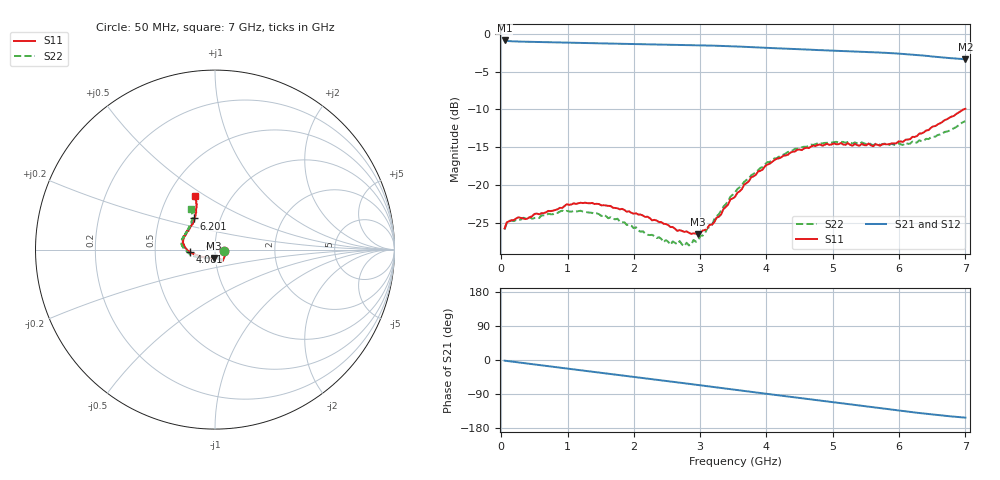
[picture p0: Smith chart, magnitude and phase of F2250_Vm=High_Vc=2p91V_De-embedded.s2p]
! Integrated Device Technology
! Corporate Headquarters
! 6024 Silver Creek Valley Road
! San Jose, CA 95138  USA
! Phone:  1-408-284-8200
! Toll Free:  1-800-223-1366
! Webpage:  http://www.idt.com/
! Timing and RF Division
! 515 Groton Road, Suite 102
! Westford, MA 01886-6024
! Device:  F2250
! Description: Voltage Variable RF Attenuator
! Frequency:  50.0 -  6000.00 MHz
! Package:  3x3 mm Thin QFN Plastic Package: 16 pin
! Ports:  2 RF, 3 DC
!  Pin  1  = GND
!  Pin  2  = NC
!  Pin  3  = RF1  = Port 1
!  Pin  4  = NC
!  Pin  5  = GND
!  Pin  6  = GND
!  Pin  7  = GND
!  Pin  8  = GND
!  Pin  9  = NC
!  Pin 10  = RF2  = Port 2
!  Pin 11  = NC
!  Pin 12  = GND
!  Pin 13  = GND
!  Pin 14  = VCNTRL
!  Pin 15  = VDD
!  Pin 16  = VMODE
! Vcntrl:  2.910 Volts
! Vmode:  +3.300 Volts
! Vdd:  +3.30  Volts
! Current:  1.315 mA
! Data:  The device was measured on a the F2250 evaluation board which has
!  individual transmission lines to the RF pins.  Data was collected
!  using a calibrated network analyzer.  The evaluation board was
!  de-embedded using a TRL calibration technique.
!  The reference plane is the edge of the package pin.
! Misc:  SN 10
!  Action Tracker AT0258
! Date Measured:  2014-11-26
! Date:  2015-10-15  MJV
! Note:
!  Integrated Device Technology supplies this data as a sample of measured
!  data at the package pin for this product.  Your particular data for this
!  product may vary.
!  Data was taken at 25 degrees C.
!  Integrated Device Technology reserves the right to change this data at anytime.
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# GHz S dB R 50
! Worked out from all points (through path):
!   201 points, 50 MHz to 7 GHz, reference 50 ohm
!   highest |S21| = -0.89 dB at 50 MHz (marker M1); lowest = -3.4 dB at 7 GHz (marker M2)
!   group delay of S21, straight-line fit = 61.2 ps
!   lowest |S11| = -26.5 dB at 2.969 GHz (marker M3), VSWR 1.10, Z = 49.1 - j4.62 ohm
!   |S11| at or under -10 dB: start of sweep to 6.967 GHz
!   |S22| runs from -28.0 to -11.5 dB; largest |S21 - S12| = 0.002
!   S11 on the Smith chart (normalised r, x): 50 MHz: 1.11, -0.02; 4.081 GHz: 0.75, -0.02; 6.201 GHz: 0.75, +0.27; 7 GHz: 0.68, +0.45
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0.05  -25.69 -10.8  -0.89 -1.8  -0.89 -1.8  -25.85 -11.0
0.1195  -24.76 -10.1  -0.99 -3.2  -0.98 -3.2  -24.69 -8.8
0.57125  -23.84 -31.3  -1.10 -13.3  -1.10 -13.3  -24.33 -31.4
0.91875  -23.00 -50.1  -1.17 -21.0  -1.17 -21.1  -23.35 -51.0
1.2315  -22.36 -57.9  -1.24 -27.9  -1.24 -27.9  -23.47 -61.5
1.75275  -23.04 -64.9  -1.33 -39.1  -1.33 -39.1  -24.42 -67.8
2.37825  -24.87 -64.5  -1.42 -52.8  -1.42 -52.8  -26.86 -66.7
2.552  -25.52 -69.4  -1.44 -56.7  -1.44 -56.7  -27.85 -73.1
2.691  -25.92 -77.5  -1.47 -59.8  -1.47 -59.8  -27.36 -80.8
2.7605  -26.16 -79.8  -1.48 -61.3  -1.48 -61.3  -28.04 -85.3
2.969  -26.49 -97.8  -1.52 -66.0  -1.52 -66.0  -27.27 -104.8
3.1775  -25.20 -120.8  -1.57 -70.7  -1.57 -70.7  -25.24 -126.7
3.525  -21.54 -152.8  -1.68 -78.5  -1.68 -78.6  -20.97 -148.7
3.76825  -18.96 -164.8  -1.77 -84.0  -1.77 -84.1  -18.70 -159.6
4.081  -16.95 -175.7  -1.90 -91.0  -1.90 -91.0  -16.72 -171.4
4.4285  -15.54 176.0  -2.03 -98.6  -2.04 -98.7  -15.20 178.7
4.7065  -14.76 169.1  -2.13 -104.8  -2.13 -104.8  -14.68 173.0
5.054  -14.61 160.9  -2.26 -112.5  -2.25 -112.5  -14.27 166.0
5.85325  -14.57 135.1  -2.56 -130.0  -2.56 -130.1  -14.67 147.3
6.20075  -13.62 123.6  -2.77 -137.7  -2.77 -137.8  -14.25 138.2
6.54825  -12.18 115.6  -3.04 -144.7  -3.04 -144.9  -13.58 126.9
7  -9.91 110.7  -3.36 -152.1  -3.37 -152.2  -11.54 120.7
